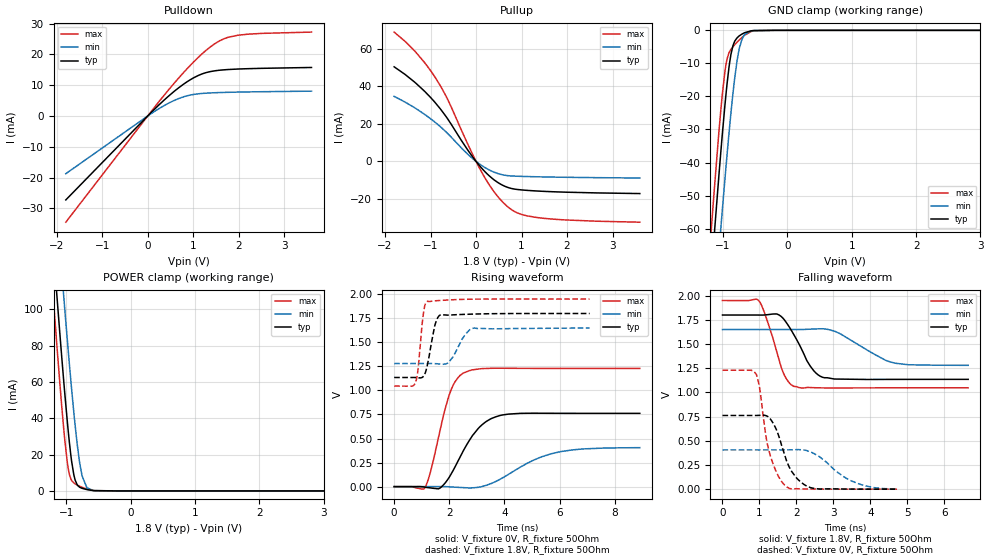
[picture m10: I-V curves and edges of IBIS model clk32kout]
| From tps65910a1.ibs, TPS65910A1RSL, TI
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|   clk32kout Model
[Model]   clk32kout
Model_type   3-state
Polarity   Non-Inverting
Vmeas = 0.9
Vref = 0
Cref = 35pF
Rref = 150
|   typ   min   max
|   (nom PVT)   (fast PVT)   (slow PVT)
C_comp   6.470e-13   6.171e-13   7.486e-13
| Where nom  PVT is Nominal Process, 1.8V, 27C
|   Fast PVT is Strong Process,  1.95V, -40C
|   Slow PVT is Weak Process,   1.65V, 125C
[Voltage Range]   1.8   1.65   1.95
|Junction Temperature
[Temperature Range]   27   125   -40
[Pullup Reference]   1.8   1.65   1.95
[Pulldown Reference]   0   0   0
[Power Clamp Reference]   1.8   1.65   1.95
[GND Clamp Reference]   0   0   0
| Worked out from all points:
|   slope of the pulldown table from 0 to 0.27 V, typ, clamps not added: 68.9 ohm
|   slope of the pullup table from 0 to 0.27 V, typ, clamps not added: 37.4 ohm
|   GND clamp passes 1 mA (typ) near -0.69 V on its own axis
|   POWER clamp passes 1 mA (typ) near -0.71 V on its own axis
|   falling waveform, V_fixture 1.8V, R_fixture 50Ohm: 20-80 % time 561ps typ, 990ps min, 435ps max; typ from 1.8 V to 1.14 V
|   rising waveform, V_fixture 0V, R_fixture 50Ohm: 20-80 % time 958ps typ, 1.63ns min, 637ps max; typ from 0 V to 0.762 V
|   rising waveform, V_fixture 1.8V, R_fixture 50Ohm: 20-80 % time 261ps typ, 424ps min, 179ps max; typ from 1.14 V to 1.8 V
|   falling waveform, V_fixture 0V, R_fixture 50Ohm: 20-80 % time 467ps typ, 854ps min, 355ps max; typ from 0.762 V to 0 V
[Pulldown]
|   Voltage   I(typ)   I(min)   I(max)
-1.8V     -27.27mA   -18.74mA   -34.5mA
150uV     2.265uA    1.538uA    2.879uA
368.4mV   5.271mA    3.439mA    6.872mA
684mV     9.199mA    5.683mA    12.38mA
900mV     11.45mA    6.684mA    15.89mA
1.154V    13.43mA    7.265mA    19.64mA
1.38V     14.44mA    7.493mA    22.48mA
1.667V    14.99mA    7.652mA    25.03mA
1.979V    15.25mA    7.761mA    26.23mA
2.508V    15.48mA    7.885mA    26.83mA
3.6V      15.76mA    8.071mA    27.25mA
[GND Clamp]
|   Voltage   I(typ)   I(min)   I(max)
-1.8V     -242.4mA   -260mA     -232.9mA
-1.182V   -73.42mA   -96.25mA   -59.94mA
-1.139V   -62.5mA    -85.56mA   -48.97mA
-1.065V   -43.95mA   -67.16mA   -30.78mA
-1.034V   -36.7mA    -59.82mA   -24.03mA
-955.8mV  -19.58mA   -41.57mA   -10.48mA
-877.7mV  -7.301mA   -25mA      -5.765mA
-846mV    -4.623mA   -19.03mA   -4.962mA
-782mV    -2.262mA   -9.146mA   -3.585mA
-707.7mV  -1.158mA   -2.805mA   -2.192mA
-520.8mV  -61.93uA   -74.41uA   -151uA
3.6V      0A         0A         0A
[Pullup]
|   Voltage   I(typ)   I(min)   I(max)
-1.8V     50.28mA    34.56mA    68.73mA
-1.322V   41.56mA    28.11mA    57.98mA
-1.108V   36.71mA    24.61mA    51.79mA
-905.7mV  31.46mA    20.91mA    44.94mA
-620.2mV  22.48mA    14.75mA    32.79mA
-180mV    5.972mA    3.772mA    9.076mA
144mV     -4.134mA   -2.496mA   -6.57mA
467.8mV   -11.03mA   -6.349mA   -18.38mA
729.1mV   -14.07mA   -7.65mA    -24.74mA
1.006V    -15.17mA   -7.961mA   -28.24mA
1.474V    -15.9mA    -8.241mA   -30.21mA
3.6V      -17.09mA   -8.824mA   -32.31mA
[POWER Clamp]
|   Voltage   I(typ)   I(min)   I(max)
-1.8V     429.9mA    472mA      410.1mA
-1.225V   143.6mA    191mA      116.6mA
-1.193V   128.8mA    176.3mA    101.6mA
-1.145V   106.3mA    153.8mA    78.83mA
-1.039V   59.61mA    106.3mA    33.35mA
-981.6mV  36.64mA    81.49mA    14.63mA
-918.6mV  16.27mA    55.99mA    5.732mA
-864mV    5.957mA    36.03mA    3.898mA
-790.2mV  1.966mA    14.75mA    2.534mA
-681.3mV  729.3uA    1.763mA    1.04mA
-565.8mV  142.7uA    187.7uA    167.8uA
3.6V      0A         0A         0A
[Ramp]
R_load = 50
|   typ   min   max
dV/dt_r   0.457076/9.56984e-10   0.243547/1.62485e-09   0.737435/6.33796e-10
dV/dt_f   0.399029/5.59816e-10   0.222251/9.84427e-10   0.541888/4.34464e-10
[Falling Waveform]
V_fixture = 1.8V
V_fixture_min = 1.65V
V_fixture_max = 1.95V
R_fixture = 50Ohm
|   Time   V(typ)   V(min)   V(max)
0s        1.8V       1.65V      1.95V
986ps     1.8V       1.65V      1.946V
1.238ns   1.804V     1.65V      1.711V
1.63ns    1.77V      1.65V      1.219V
1.936ns   1.594V     1.65V      1.062V
2.376ns   1.272V     1.654V     1.05V
2.714ns   1.156V     1.658V     1.047V
3.196ns   1.137V     1.605V     1.046V
4.552ns   1.134V     1.314V     1.047V
6.65ns    1.135V     1.28V      1.047V
[Rising Waveform]
V_fixture = 0V
V_fixture_min = 0V
V_fixture_max = 0V
R_fixture = 50Ohm
|   Time   V(typ)   V(min)   V(max)
0s        257.2pV    515.3pV    248.8pV
1.112ns   -5.661mV   -398nV     -14.12mV
1.314ns   -13.51mV   -11.37uV   148.8mV
1.602ns   -23.42mV   326.3uV    503.4mV
1.996ns   96.81mV    -1.897mV   952.6mV
2.512ns   374.3mV    -10.39mV   1.181V
3.16ns    635.8mV    -1.023mV   1.226V
3.914ns   744.2mV    87.9mV     1.231V
6.054ns   762.2mV    364.6mV    1.229V
8.91ns    761.8mV    405.3mV    1.229V
[Rising Waveform]
V_fixture = 1.8V
V_fixture_min = 1.65V
V_fixture_max = 1.95V
R_fixture = 50Ohm
|   Time   V(typ)   V(min)   V(max)
0s        1.135V     1.28V      1.045V
770ps     1.135V     1.28V      1.078V
868ps     1.132V     1.28V      1.224V
1.072ns   1.151V     1.28V      1.82V
1.206ns   1.265V     1.28V      1.927V
1.47ns    1.668V     1.279V     1.931V
1.694ns   1.788V     1.274V     1.936V
1.99ns    1.783V     1.297V     1.941V
2.824ns   1.793V     1.644V     1.949V
7.09ns    1.8V       1.65V      1.95V
[Falling Waveform]
V_fixture = 0V
V_fixture_min = 0V
V_fixture_max = 0V
R_fixture = 50Ohm
|   Time   V(typ)   V(min)   V(max)
0s        761.8mV    405.9mV    1.229V
918ps     761.7mV    405.9mV    1.184V
1.024ns   763.5mV    405.9mV    998.2mV
1.176ns   759.8mV    405.9mV    546.5mV
1.298ns   723.9mV    405.9mV    341.7mV
1.738ns   288.7mV    405.9mV    23.76mV
2.024ns   107.6mV    408.6mV    4.414mV
2.392ns   14.72mV    384mV      1.876mV
3.458ns   648.9uV    90.27mV    -139.6uV
4.738ns   19.14uV    213.5uV    20.68uV
